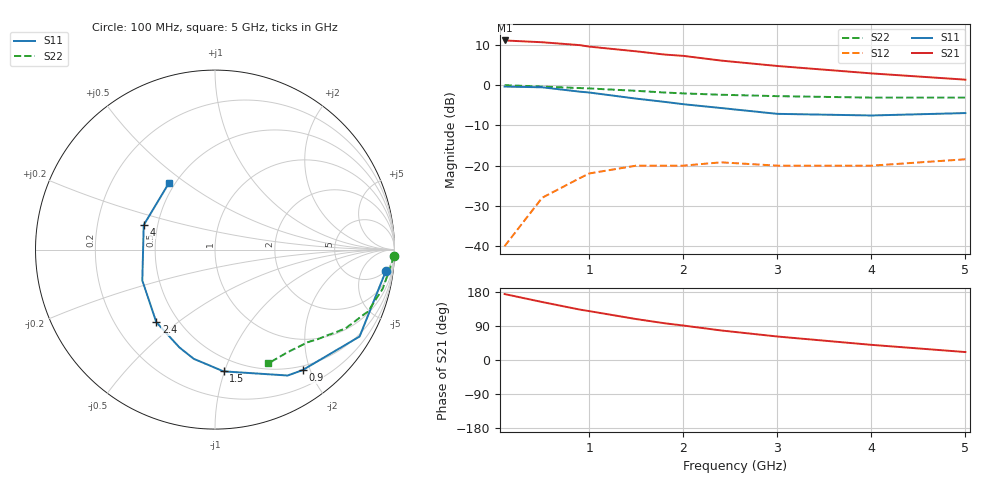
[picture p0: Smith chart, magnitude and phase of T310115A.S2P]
!AT-31011
!S and NOISE PARAMETERS at Vce=5V  Ic=1mA.  LAST UPDATED 06-23-94
# ghz s ma r 50
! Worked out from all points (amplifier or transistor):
!   11 points, 100 MHz to 5 GHz, reference 50 ohm
!   highest |S21| = 11.1 dB at 100 MHz (marker M1)
!   |S21| within 3 dB of that: start of sweep to 1.612 GHz
!   unconditionally stable (mu >= 1): 2.897 GHz to end of sweep
!   at 500 MHz: K = 0.16, MSG = 19.3 dB, |S12| = -28.0 dB
!   at 1.8 GHz: K = 0.58, MSG = 13.8 dB, |S12| = -20.0 dB
!   at 5 GHz: K = 1.20, MAG = 7.2 dB, |S12| = -18.4 dB
!   lowest NFmin = 0.50 dB at 500 MHz
!   S11 on the Smith chart (normalised r, x): 100 MHz: 5, -15; 900 MHz: 0.44, -1.88; 1.5 GHz: 0.39, -0.99; 2.4 GHz: 0.38, -0.42; 4 GHz: 0.42, +0.14; 5 GHz: 0.46, +0.43
0.1  0.96 -7.0  3.59 174.0  0.01 84.0  0.999 -2.0
0.5  0.94 -31.0  3.41 153.0  0.04 69.0  0.96 -13.0
0.9  0.83 -54.0  3.14 133.0  0.07 56.0  0.92 -22.0
1  0.81 -60.0  3.01 129.0  0.08 53.0  0.91 -23.0
1.5  0.68 -86.0  2.63 108.0  0.1 41.0  0.85 -31.0
1.8  0.62 -101.0  2.4 97.0  0.1 35.0  0.81 -35.0
2  0.58 -110.0  2.31 91.0  0.1 32.0  0.79 -37.0
2.4  0.52 -129.0  2.02 78.0  0.11 28.0  0.76 -41.0
3  0.44 -157.0  1.73 62.0  0.1 26.0  0.73 -45.0
4  0.42 161.0  1.4 40.0  0.1 31.0  0.7 -55.0
5  0.45 125.0  1.17 21.0  0.12 43.0  0.7 -65.0
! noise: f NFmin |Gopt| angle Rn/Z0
0.5  0.5  0.92  13  0.85
0.9  0.6  0.85  29  0.73
1.8  1.1  0.68  67  0.46
2.4  1.6  0.55  98  0.28
